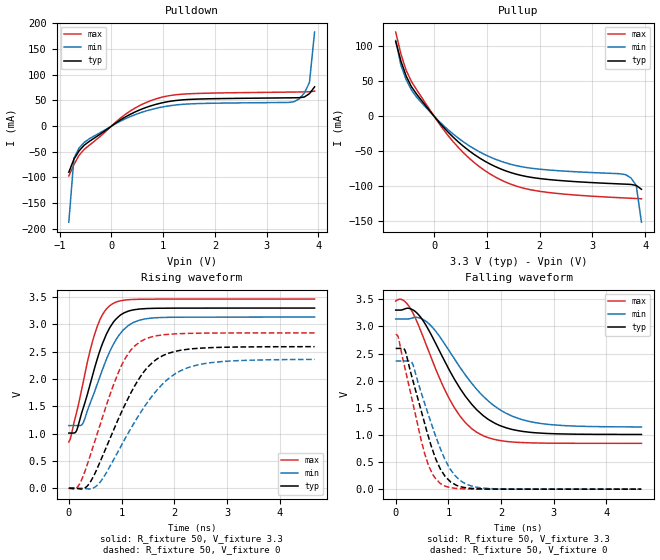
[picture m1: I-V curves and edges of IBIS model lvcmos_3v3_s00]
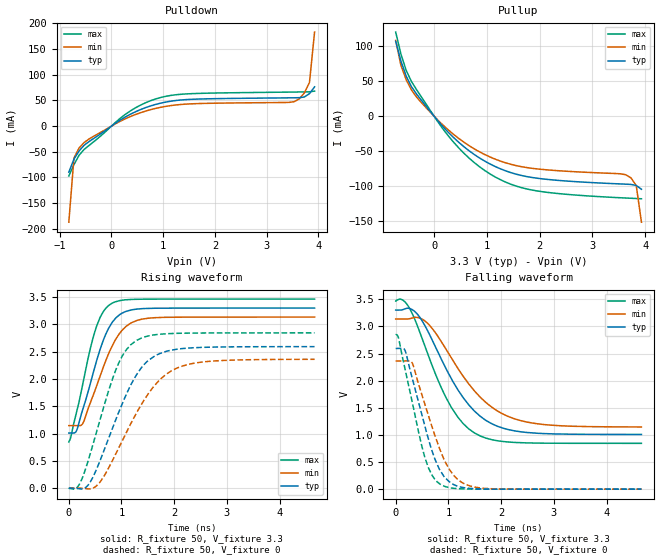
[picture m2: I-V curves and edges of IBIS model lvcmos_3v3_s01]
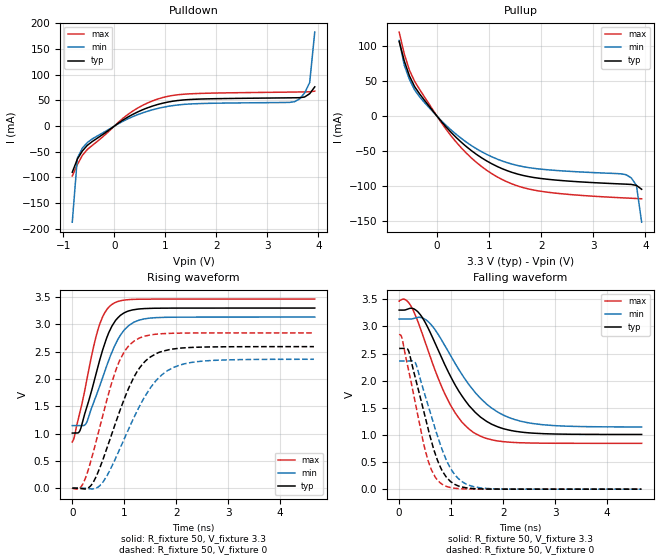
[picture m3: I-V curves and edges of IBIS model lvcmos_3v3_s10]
[IBIS ver]   4.1
[File name]   5p49v5907.ibs
[File Rev]   1.0
[Date]   May 27, 2015
[Source]   IDT
[Notes]   1. Temp typ=25C, min=85C, max=-40C
[Disclaimer]
READ THESE TERMS AND CONDITIONS CAREFULLY BEFORE USING THIS IBIS MODEL.  BY
USING THIS IBIS MODEL, YOU ARE ACCEPTING AND AGREEING TO THESE TERMS AND
CONDITIONS OF USE.
INTEGRATED DEVICE TECHNOLOGY, INC. ("IDT") HEREBY GRANTS THE USER OF THIS
IBIS MODEL ("USER") A NON-EXCLUSIVE, NONTRANSFERABLE LICENSE TO USE THIS
IBIS MODEL UNDER THE FOLLOWING TERMS: THE USER IS GRANTED THIS LICENSE ONLY
TO USE THE IBIS MODEL FOR DEMONSTRATION PURPOSES ONLY AND IS NOT GRANTED
RIGHTS TO SELL, COPY (EXCEPT AS NEEDED TO RUN THE IBIS MODEL), RENT, LEASE
OR SUB-LICENSE (EXCEPT FOR DEMONSTRATION) THE IBIS MODEL IN WHOLE OR IN
PART, OR IN MODIFIED FORM TO ANYONE. THE USER MAY MODIFY THE IBIS MODEL TO
SUIT ITS SPECIFIC APPLICATIONS, BUT  RIGHTS TO DERIVATIVE WORKS AND SUCH
MODIFICATIONS SHALL BELONG TO IDT.
THIS IBIS MODEL IS PROVIDED ON AN AS IS" BASIS AND IDT  MAKES ABSOLUTELY NO
WARRANTY WITH RESPECT TO THE INFORMATION CONTAINED HEREIN.  IDT DISCLAIMS
AND USER WAIVES ALL WARRANTIES, EXPRESS AND IMPLIED, INCLUDING WARRANTIES OF
MERCHANTABILITY AND FITNESS FOR A PARTICULAR PURPOSE.  THE ENTIRE RISK AS TO
QUALITY AND PERFORMANCE IS WITH THE USER  ACCORDINGLY, IN NO EVENT SHALL IDT
BE LIABLE FOR ANY DIRECT OR INDIRECT DAMAGES, WHETHER IN CONTRACT OR TORT,
INCLUDING ANY LOST PROFITS OR OTHER INCIDENTAL, CONSEQUENTIAL, EXEMPLARY, OR
PUNITIVE DAMAGES ARISING OUT OF THE USE OR APPLICATION OF THE  IBIS MODEL,
WHETHER OR NOT IDT HAD NOTICE OF SUCH DAMAGES.
IDT RESERVES THE RIGHT TO MAKE CHANGES WITHOUT NOTICE TO ANY PRODUCT HEREIN
TO IMPROVE RELIABILITY, FUNCTION, OR DESIGN. IDT DOES NOT CONVEY ANY LICENSE
UNDER PATENT RIGHTS OR ANY OTHER INTELLECTUAL PROPERTY RIGHTS, INCLUDING
THOSE OF THIRD PARTIES. IDT IS NOT OBLIGATED TO PROVIDE  MAINTENANCE OR
SUPPORT FOR THE LICENSED IBIS MODEL.
This model is for  vc5 IDT Programmable Clock
[Copyright]
Copyright 2002, Integrated Device Technology, Inc. All rights  reserved.
|History
|Rev 1.0 Created on May 27, 2015
|   Component IDT5p49v5907
[Component]   IDT5V49V5907
[Manufacturer]   Integrated Device Technology Inc.
[Package]
| Following package parameters are for the 24 pin QFN package
| variable   typ   min   max
R_pkg   72.4655m   58.886m   86.045m
L_pkg   1.47175nH   1.11650nH   1.77850nH
C_pkg   0.07747pF   0.07444pF   0.08050pF
[Pin]  signal_name   model_name
1   NC   NC
2   XOUT   NC
3   XIN/REF   input
4   VDDA   POWER
5   VDDO   POWER
6   OUT7   LP_HCSL
7   OUT7B   LP_HCSL
8   OUT6   LP_HCSL
9   OUT6B   LP_HCSL
10   SD/OE   input
11   SEL1/SDA   input
12   SEL0/SCL   input
13   VDD   POWER
14   VDDO   POWER
15   OUT5   LP_HCSL
16   OUT5B   LP_HCSL
17   OEB35   input
18   VDDO4   POWER
19   OUT4   UIO
20   OUT4B   UIO
21   NC   NC
22   NC   NC
23   OUT3B   LP_HCSL
24   OUT3   LP_HCSL
25   VDD_CORE   POWER
26   VDD   POWER
27   VDD   POWER
28   OUT2B   UIO
29   OUT2   UIO
30   VDDO2   POWER
31   OUT1B   UIO
32   OUT1   UIO
33   VDDO1   POWER
34   OEB67   input
35   NC   NC
36   VDDO   POWER
37   VDD   POWER
38   OEBUFFER   input
39   VDDO0   POWER
40   OUT0_SEL_I2C   UIOLVCMOS
[Diff Pin]  inv_pin  vdiff   tdelay_typ  tdelay_min  tdelay_max
|1   2   0.000V   0.000s   0.000s   0.000s
6   7   0.000V   0.000s   0.000s   0.000s
8   9   0.000V   0.000s   0.000s   0.000s
15   16   0.000V   0.000s   0.000s   0.000s
19   20   0.000V   0.000s   0.000s   0.000s
24   23   0.000V   0.000s   0.000s   0.000s
29   28   0.000V   0.000s   0.000s   0.000s
32   31   0.000V   0.000s   0.000s   0.000s
[Model Selector] UIO
lvcmos_3v3_s00 slew rate 00
lvcmos_3v3_s01 slew rate 01
lvcmos_3v3_s10 slew rate 10
lvcmos_3v3_s11 slew rate 11
lvcmos_2v5_s00 slew rate 00
lvcmos_2v5_s01 slew rate 01
lvcmos_2v5_s10 slew rate 10
lvcmos_2v5_s11 slew rate 11
lvcmos_1v8_s00 slew rate 00
lvcmos_1v8_s01 slew rate 01
lvcmos_1v8_s10 slew rate 10
lvcmos_1v8_s11 slew rate 11
hcsl_3v3 slew rate 11
hcsl_2v5 slew rate 11
lvds_3v3  slew rate 11
lvds_2v5  slew rate 11
lvpecl_3v3 slew rate 11
lvpecl_2v5 slew rate 11
[Model Selector] UIOLVCMOS
lvcmos_3v3_s00 slew rate 00
lvcmos_3v3_s01 slew rate 01
lvcmos_3v3_s10 slew rate 10
lvcmos_3v3_s11 slew rate 11
lvcmos_2v5_s00 slew rate 00
lvcmos_2v5_s01 slew rate 01
lvcmos_2v5_s10 slew rate 10
lvcmos_2v5_s11 slew rate 11
lvcmos_1v8_s00 slew rate 00
lvcmos_1v8_s01 slew rate 01
lvcmos_1v8_s10 slew rate 10
lvcmos_1v8_s11 slew rate 11
| Models and submodels in the file (20): lvcmos_3v3_s00 (Output), lvcmos_3v3_s01 (Output), lvcmos_3v3_s10 (Output), lvcmos_3v3_s11 (Output), lvcmos_2v5_s00 (Output), lvcmos_2v5_s01 (Output), lvcmos_2v5_s10 (Output), lvcmos_2v5_s11 (Output), lvcmos_1v8_s00 (Output), lvcmos_1v8_s01 (Output), lvcmos_1v8_s10 (Output), lvcmos_1v8_s11 (Output), hcsl_3v3 (Open_source), hcsl_2v5 (Open_source), lvds_3v3 (Output), lvds_2v5 (Output), lvpecl_3v3 (Output_ECL), lvpecl_2v5 (Output_ECL), LP_HCSL (Output), input (Input)
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|   Model LVCMOS_3V3
[Model]   lvcmos_3v3_s00
Model_type   Output
Polarity   Non-Inverting
|   typ   min   max
C_comp   2pF   1.5pF   2.5pF
Vmeas = 1.65V
Rref = 50
Cref = 0
Vref = 1.65V
|   typ   min   max
[Voltage range]   3.3V   3.135V   3.465V
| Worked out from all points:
|   slope of the pulldown table from 0 to 0.495 V, typ, clamps not added: 16.9 ohm
|   slope of the pullup table from 0 to 0.495 V, typ, clamps not added: 12.6 ohm
|   rising waveform, R_fixture 50, V_fixture 3.3: 20-80 % time 450ps typ, 507ps min, 388ps max; typ from 1.01 V to 3.3 V
|   falling waveform, R_fixture 50, V_fixture 3.3: 20-80 % time 857ps typ, 970ps min, 739ps max; typ from 3.3 V to 1.01 V
|   rising waveform, R_fixture 50, V_fixture 0: 20-80 % time 771ps typ, 936ps min, 618ps max; typ from 0 V to 2.59 V
|   falling waveform, R_fixture 50, V_fixture 0: 20-80 % time 472ps typ, 527ps min, 413ps max; typ from 2.59 V to 0 V
[Pulldown]
|Voltage   I (typ)   I (min)   I (max)
|Note, modeling breaks down at 250mA and above.  This is well beyond the functional   |
|operating range of the device.  Should this scenario occur, catastrophic failure and   |
|possible damage to the device and/or board is of higher concern than the I-V curve   |
|behavior.  The IBIS checker will flag currents in excess of 10A with warnings.  Lines   |
|with currents in excess of 0.35 A have been commented out.  The points still remain|
|available to the user if the user desires to use them.   |
|-3.30000e+00   -4.58626e+02   -3.98855e+02   -5.58913e+02
|-3.20100e+00   -4.38670e+02   -3.81813e+02   -5.34126e+02
|-3.10200e+00   -4.18718e+02   -3.64776e+02   -5.09343e+02
|-3.00300e+00   -3.98770e+02   -3.47745e+02   -4.84563e+02
|-2.90400e+00   -3.78827e+02   -3.30720e+02   -4.59787e+02
|-2.80500e+00   -3.58890e+02   -3.13701e+02   -4.35015e+02
|-2.70600e+00   -3.38959e+02   -2.96690e+02   -4.10248e+02
|-2.60700e+00   -3.19035e+02   -2.79688e+02   -3.85486e+02
|-2.50800e+00   -2.99119e+02   -2.62696e+02   -3.60731e+02
|-2.40900e+00   -2.79213e+02   -2.45715e+02   -3.35984e+02
|-2.31000e+00   -2.59319e+02   -2.28747e+02   -3.11245e+02
|-2.21100e+00   -2.39437e+02   -2.11796e+02   -2.86516e+02
|-2.11200e+00   -2.19572e+02   -1.94864e+02   -2.61800e+02
|-2.01300e+00   -1.99726e+02   -1.77955e+02   -2.37100e+02
|-1.91400e+00   -1.79905e+02   -1.61075e+02   -2.12419e+02
|-1.81500e+00   -1.60116e+02   -1.44233e+02   -1.87763e+02
|-1.71600e+00   -1.40369e+02   -1.27441e+02   -1.63140e+02
|-1.61700e+00   -1.20682e+02   -1.10717e+02   -1.38565e+02
|-1.51800e+00   -1.01080e+02   -9.40899e+01   -1.14061e+02
|-1.41900e+00   -8.16135e+01   -7.76121e+01   -8.96701e+01
|-1.32000e+00   -6.23864e+01   -6.13830e+01   -6.54941e+01
|-1.22100e+00   -4.36066e+01   -4.55730e+01   -4.17841e+01
|-1.12200e+00   -2.55446e+01   -3.03740e+01   -1.89497e+01
|-1.02300e+00   -8.13369e+00   -1.57511e+01   -1.01906e+00
|-9.24000e-01   -3.55892e-01   -2.38948e+00   -1.27879e-01
-825mV    -89.74mA   -186.9mA   -97.05mA
-726mV    -64.34mA   -62.46mA   -75.03mA
-627mV    -48.3mA    -42.65mA   -56.86mA
-528mV    -37.22mA   -31.89mA   -45.33mA
363mV     22.88mA    18.45mA    29.33mA
957mV     44.74mA    36.62mA    55.73mA
1.551V    52.05mA    43.3mA     63.04mA
3.531V    55.03mA    47.39mA    66.19mA
3.63V     55.21mA    52.95mA    66.32mA
3.729V    56.59mA    64.36mA    66.46mA
3.828V    63.02mA    84.81mA    66.64mA
3.927V    76.26mA    182.8mA    67.99mA
| 4.02600e+00   9.63336e-02   1.95544e+00   7.56685e-02
| 4.12500e+00   1.29319e-01   1.96109e+01   9.19025e-02
| 4.22400e+00   6.62462e-01   4.21550e+01   1.15435e-01
| 4.32300e+00   1.51637e+01   6.47670e+01   1.37492e-01
| 4.42200e+00   4.22442e+01   8.74545e+01   2.35006e-01
| 4.52100e+00   6.94172e+01   1.10195e+02   8.92943e+00
| 4.62000e+00   9.66780e+01   1.32968e+02   4.35589e+01
| 4.71900e+00   1.23991e+02   1.55761e+02   7.83218e+01
| 4.81800e+00   1.51333e+02   1.78569e+02   1.13180e+02
| 4.91700e+00   1.78693e+02   2.01386e+02   1.48085e+02
| 5.01600e+00   2.06065e+02   2.24210e+02   1.83014e+02
| 5.11500e+00   2.33446e+02   2.47041e+02   2.17958e+02
| 5.21400e+00   2.60834e+02   2.69877e+02   2.52912e+02
| 5.31300e+00   2.88228e+02   2.92717e+02   2.87874e+02
| 5.41200e+00   3.15625e+02   3.15560e+02   3.22841e+02
| 5.51100e+00   3.43027e+02   3.38407e+02   3.57813e+02
| 5.61000e+00   3.70432e+02   3.61256e+02   3.92789e+02
| 5.70900e+00   3.97841e+02   3.84108e+02   4.27769e+02
| 5.80800e+00   4.25252e+02   4.06963e+02   4.62752e+02
| 5.90700e+00   4.52666e+02   4.29821e+02   4.97738e+02
| 6.00600e+00   4.80082e+02   4.52680e+02   5.32727e+02
| 6.10500e+00   5.07501e+02   4.75543e+02   5.67718e+02
| 6.20400e+00   5.34922e+02   4.98407e+02   6.02711e+02
| 6.30300e+00   5.62345e+02   5.21273e+02   6.37705e+02
| 6.40200e+00   5.89770e+02   5.44142e+02   6.72701e+02
| 6.50100e+00   6.17197e+02   5.67013e+02   7.07699e+02
| 6.60000e+00   6.44626e+02   5.89886e+02   7.42698e+02
[Pullup]
|Voltage   I (typ)   I (min)   I (max)
|Note, modeling breaks down at 250mA and above.  This is well beyond the functional   |
|operating range of the device.  Should this scenario occur, catastrophic failure and   |
|possible damage to the device and/or board is of higher concern than the I-V curve   |
|behavior.  The IBIS checker will flag currents in excess of 10A with warnings.  Lines   |
|with currents in excess of 0.35 A have been commented out.  The points still remain|
|available to the user if the user desires to use them.   |
|-3.30000e+00   6.44680e+02   5.51825e+02   8.01095e+02
|-3.20100e+00   6.17254e+02   5.28958e+02   7.66095e+02
|-3.10200e+00   5.89830e+02   5.06093e+02   7.31096e+02
|-3.00300e+00   5.62407e+02   4.83230e+02   6.96098e+02
|-2.90400e+00   5.34987e+02   4.60368e+02   6.61102e+02
|-2.80500e+00   5.07568e+02   4.37509e+02   6.26108e+02
|-2.70600e+00   4.80150e+02   4.14651e+02   5.91115e+02
|-2.60700e+00   4.52735e+02   3.91796e+02   5.56124e+02
|-2.50800e+00   4.25322e+02   3.68942e+02   5.21136e+02
|-2.40900e+00   3.97911e+02   3.46091e+02   4.86149e+02
|-2.31000e+00   3.70503e+02   3.23243e+02   4.51165e+02
|-2.21100e+00   3.43097e+02   3.00397e+02   4.16183e+02
|-2.11200e+00   3.15694e+02   2.77554e+02   3.81204e+02
|-2.01300e+00   2.88295e+02   2.54715e+02   3.46229e+02
|-1.91400e+00   2.60900e+02   2.31881e+02   3.11257e+02
|-1.81500e+00   2.33510e+02   2.09052e+02   2.76290e+02
|-1.71600e+00   2.06127e+02   1.86229e+02   2.41329e+02
|-1.61700e+00   1.78751e+02   1.63415e+02   2.06375e+02
|-1.51800e+00   1.51388e+02   1.40613e+02   1.71432e+02
|-1.41900e+00   1.24042e+02   1.17829e+02   1.36506e+02
|-1.32000e+00   9.67252e+01   9.50724e+01   1.01609e+02
|-1.22100e+00   6.94599e+01   7.23604e+01   6.67700e+01
|-1.12200e+00   4.22820e+01   4.97173e+01   3.20469e+01
|-1.02300e+00   1.51962e+01   2.71494e+01   2.11287e+00
|-9.24000e-01   6.89030e-01   5.34223e+00   1.97623e-01
|-8.25000e-01   1.48916e-01   3.54714e-01   1.54087e-01
-726mV    106.9mA    108.2mA    120.1mA
-627mV    78.63mA    72.64mA    88.74mA
-528mV    57.36mA    52.3mA     65.5mA
-330mV    31.45mA    27.24mA    37.82mA
363mV     -30.02mA   -25.58mA   -36.52mA
957mV     -64.05mA   -54.65mA   -77.43mA
1.353V    -77.99mA   -66.51mA   -94.06mA
1.848V    -87.45mA   -74.38mA   -105.4mA
3.63V     -97.08mA   -83.63mA   -116.9mA
3.729V    -97.47mA   -88.18mA   -117.2mA
3.828V    -98.9mA    -99mA      -117.5mA
3.927V    -104.4mA   -151.4mA   -117.9mA
| 4.02600e+00   -1.15410e-01   -9.65481e-01   -1.19366e-01
| 4.12500e+00   -1.36603e-01   -1.09884e+01   -1.26324e-01
| 4.22400e+00   -3.99361e-01   -2.54841e+01   -1.40663e-01
| 4.32300e+00   -8.17474e+00   -4.04654e+01   -1.58277e-01
| 4.42200e+00   -2.55843e+01   -5.60873e+01   -2.17491e-01
| 4.52100e+00   -4.36450e+01   -7.21990e+01   -4.28595e+00
| 4.62000e+00   -6.24226e+01   -8.86071e+01   -2.64922e+01
| 4.71900e+00   -8.16508e+01   -1.05189e+02   -4.96573e+01
| 4.81800e+00   -1.01115e+02   -1.21884e+02   -7.35635e+01
| 4.91700e+00   -1.20715e+02   -1.38656e+02   -9.78285e+01
| 5.01600e+00   -1.40403e+02   -1.55482e+02   -1.22263e+02
| 5.11500e+00   -1.60149e+02   -1.72350e+02   -1.46794e+02
| 5.21400e+00   -1.79938e+02   -1.89250e+02   -1.71387e+02
| 5.31300e+00   -1.99760e+02   -2.06175e+02   -1.96022e+02
| 5.41200e+00   -2.19606e+02   -2.23121e+02   -2.20688e+02
| 5.51100e+00   -2.39472e+02   -2.40084e+02   -2.45378e+02
| 5.61000e+00   -2.59355e+02   -2.57061e+02   -2.70086e+02
| 5.70900e+00   -2.79251e+02   -2.74051e+02   -2.94808e+02
| 5.80800e+00   -2.99159e+02   -2.91052e+02   -3.19543e+02
| 5.90700e+00   -3.19077e+02   -3.08062e+02   -3.44288e+02
| 6.00600e+00   -3.39003e+02   -3.25080e+02   -3.69042e+02
| 6.10500e+00   -3.58937e+02   -3.42106e+02   -3.93803e+02
| 6.20400e+00   -3.78878e+02   -3.59138e+02   -4.18571e+02
| 6.30300e+00   -3.98826e+02   -3.76177e+02   -4.43346e+02
| 6.40200e+00   -4.18779e+02   -3.93221e+02   -4.68125e+02
| 6.50100e+00   -4.38737e+02   -4.10271e+02   -4.92910e+02
| 6.60000e+00   -4.58699e+02   -4.27325e+02   -5.17700e+02
[Ramp]
|   typ   min   max
dV/dt_r   1.566/0.774n   1.425/0.94n   1.718/0.621n
dV/dt_f   1.396/0.866n   1.212/0.979n   1.595/0.746n
R_load =   50
[Rising Waveform]
R_fixture = 50
V_fixture = 3.3   |Vcc_typ
V_fixture_min = 3.135 |Vcc_min
V_fixture_max = 3.465 |Vcc_max
C_fixture = 0.0p
| Time   typ   min   max
| 0.00000e+00   1.00813e+00   1.14515e+00   8.44568e-01
| 2.69541e-12   1.00813e+00   1.14515e+00   8.44568e-01
| 4.88539e-12   1.00813e+00   1.14515e+00   8.44568e-01
| 5.15560e-12   1.00813e+00   1.14515e+00   8.44568e-01
| 8.43814e-12   1.00813e+00   1.14515e+00   8.44568e-01
| 1.48885e-11   1.00813e+00   1.14515e+00   8.44568e-01
| 1.56443e-11   1.00813e+00   1.14515e+00   8.44568e-01
| 2.89352e-11   1.00813e+00   1.14515e+00   8.44568e-01
| 4.35521e-11   1.00813e+00   1.14515e+00   8.44568e-01
| 4.98146e-11   1.00813e+00   1.14515e+00   8.44568e-01
| 5.87208e-11   1.00813e+00   1.14515e+00   8.44568e-01
| 7.00000e-11   1.00813e+00   1.14515e+00   8.44568e-01
| 7.43355e-11   1.00813e+00   1.14515e+00   8.44568e-01
| 7.98941e-11   1.00813e+00   1.14515e+00   8.44568e-01
| 8.04812e-11   1.00813e+00   1.14515e+00   8.44568e-01
| 8.54765e-11   1.00813e+00   1.14515e+00   8.44568e-01
| 9.54712e-11   1.00813e+00   1.14515e+00   8.44568e-01
| 9.66941e-11   1.00813e+00   1.14515e+00   8.44568e-01
| 1.09694e-10   1.00813e+00   1.14515e+00   8.44568e-01
| 1.16904e-10   1.00813e+00   1.14515e+00   8.44568e-01
| 1.22050e-10   1.00813e+00   1.14515e+00   8.44568e-01
| 1.33756e-10   1.00813e+00   1.14515e+00   8.44568e-01
| 1.42319e-10   1.00813e+00   1.14515e+00   8.44568e-01
| 1.49876e-10   1.00813e+00   1.14515e+00   8.44568e-01
| 1.59675e-10   1.00813e+00   1.14515e+00   8.44568e-01
| 1.71924e-10   1.00813e+00   1.14515e+00   8.44568e-01
| 1.80502e-10   1.00813e+00   1.14515e+00   8.44568e-01
| 1.93342e-10   1.00813e+00   1.14515e+00   8.44568e-01
| 2.03187e-10   1.00813e+00   1.14515e+00   8.44568e-01
| 2.12788e-10   1.00813e+00   1.14515e+00   8.44568e-01
| 2.20117e-10   1.00813e+00   1.14515e+00   8.44568e-01
| 2.25959e-10   1.00813e+00   1.14515e+00   8.44568e-01
| 2.28188e-10   1.00813e+00   1.14515e+00   8.44568e-01
| 2.36412e-10   1.00813e+00   1.14515e+00   8.44568e-01
| 2.43714e-10   1.00813e+00   1.14515e+00   8.44568e-01
| 2.46567e-10   1.00813e+00   1.14515e+00   8.44568e-01
| 2.54564e-10   1.00813e+00   1.14515e+00   8.44568e-01
| 2.64894e-10   1.00813e+00   1.14515e+00   8.44568e-01
| 2.65919e-10   1.00813e+00   1.14515e+00   8.44568e-01
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0s        1.008V     1.145V     844.6mV
34.71ps   1.008V     1.145V     923.1mV
154.3ps   1.071V     1.145V     1.413V
275.2ps   1.472V     1.202V     1.956V
479.5ps   2.168V     1.745V     2.789V
635.5ps   2.641V     2.166V     3.174V
823.7ps   3.01V      2.596V     3.375V
1.129ns   3.244V     2.981V     3.453V
1.433ns   3.289V     3.099V     3.463V
4.662ns   3.3V       3.135V     3.465V
[Falling Waveform]
R_fixture = 50
V_fixture = 3.3   |Vcc_typ
V_fixture_min = 3.135 |Vcc_min
V_fixture_max = 3.465 |Vcc_max
C_fixture = 0.0p
| Time   typ   min   max
| 0.00000e+00   3.30000e+00   3.13500e+00   3.46500e+00
| 2.69541e-12   3.30000e+00   3.13500e+00   3.46500e+00
| 4.88539e-12   3.30000e+00   3.13500e+00   3.46500e+00
| 5.15560e-12   3.30000e+00   3.13500e+00   3.46500e+00
| 8.43814e-12   3.30000e+00   3.13500e+00   3.46500e+00
| 1.48885e-11   3.30000e+00   3.13500e+00   3.46500e+00
| 1.56443e-11   3.30000e+00   3.13500e+00   3.46500e+00
| 2.89352e-11   3.30000e+00   3.13500e+00   3.46500e+00
| 4.35521e-11   3.30000e+00   3.13500e+00   3.46500e+00
| 4.98146e-11   3.30000e+00   3.13500e+00   3.46500e+00
| 5.87207e-11   3.30000e+00   3.13500e+00   3.46500e+00
| 7.00000e-11   3.30000e+00   3.13500e+00   3.46500e+00
| 7.43355e-11   3.30000e+00   3.13500e+00   3.46500e+00
| 7.98941e-11   3.30000e+00   3.13500e+00   3.46500e+00
| 8.04812e-11   3.30000e+00   3.13500e+00   3.46500e+00
| 8.54765e-11   3.30000e+00   3.13500e+00   3.46500e+00
| 9.54712e-11   3.30000e+00   3.13500e+00   3.46500e+00
| 9.66941e-11   3.30000e+00   3.13500e+00   3.46500e+00
| 1.09694e-10   3.30000e+00   3.13500e+00   3.46500e+00
| 1.16904e-10   3.30000e+00   3.13500e+00   3.46500e+00
| 1.22050e-10   3.30000e+00   3.13500e+00   3.46500e+00
| 1.33756e-10   3.30000e+00   3.13500e+00   3.46500e+00
| 1.42318e-10   3.30000e+00   3.13500e+00   3.46500e+00
| 1.49875e-10   3.30000e+00   3.13500e+00   3.46500e+00
| 1.59673e-10   3.30000e+00   3.13500e+00   3.46500e+00
| 1.72937e-10   3.30000e+00   3.13500e+00   3.46500e+00
| 1.80499e-10   3.30000e+00   3.13500e+00   3.46500e+00
| 1.94084e-10   3.30000e+00   3.13500e+00   3.46500e+00
| 2.03953e-10   3.30000e+00   3.13500e+00   3.46500e+00
| 2.17182e-10   3.30000e+00   3.13500e+00   3.46500e+00
| 2.22997e-10   3.30000e+00   3.13500e+00   3.46500e+00
| 2.32435e-10   3.30000e+00   3.13500e+00   3.46500e+00
| 2.41161e-10   3.30000e+00   3.13500e+00   3.46500e+00
| 2.46386e-10   3.30000e+00   3.13500e+00   3.46500e+00
| 2.56120e-10   3.30000e+00   3.13500e+00   3.46500e+00
| 2.57140e-10   3.30000e+00   3.13500e+00   3.46500e+00
| 2.66989e-10   3.30000e+00   3.13500e+00   3.46500e+00
| 2.77410e-10   3.30000e+00   3.13500e+00   3.46500e+00
| 2.83433e-10   3.30000e+00   3.13500e+00   3.46500e+00
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0s        3.3V       3.135V     3.465V
120.3ps   3.304V     3.135V     3.493V
247.8ps   3.333V     3.138V     3.377V
425ps     3.225V     3.162V     3.038V
624.4ps   2.937V     3.054V     2.545V
1.111ns   2.034V     2.407V     1.506V
1.539ns   1.462V     1.838V     1.048V
1.979ns   1.171V     1.463V     896.3mV
2.515ns   1.052V     1.252V     854.4mV
4.666ns   1.008V     1.146V     844.6mV
[Rising Waveform]
R_fixture = 50
V_fixture = 0
C_fixture = 0.0p
| Time   typ   min   max
| 0.00000e+00   2.38922e-08   6.04307e-08   3.04013e-08
| 2.76195e-12   2.38928e-08   6.04313e-08   3.04019e-08
| 5.02196e-12   2.38933e-08   6.04317e-08   3.04024e-08
| 8.43814e-12   2.38939e-08   6.04323e-08   3.04029e-08
| 1.48885e-11   2.38940e-08   6.04329e-08   3.04024e-08
| 2.82261e-11   2.38916e-08   6.04313e-08   3.03997e-08
| 2.96292e-11   2.38914e-08   6.04311e-08   3.03993e-08
| 4.65264e-11   2.38885e-08   6.04278e-08   3.03985e-08
| 5.82632e-11   2.38858e-08   6.04236e-08   3.03966e-08
| 5.99073e-11   2.38849e-08   6.04221e-08   3.03962e-08
| 7.43093e-11   2.38731e-08   6.04054e-08   3.03887e-08
| 7.44096e-11   2.38730e-08   6.04053e-08   3.03887e-08
| 8.01162e-11   2.38724e-08   6.03982e-08   3.03965e-08
| 8.50865e-11   2.38893e-08   6.04041e-08   3.04290e-08
| 8.58855e-11   2.38922e-08   6.04086e-08   3.04412e-08
| 9.61972e-11   2.40299e-08   6.05121e-08   3.05978e-08
| 1.07592e-10   2.42393e-08   6.07310e-08   3.07509e-08
| 1.10532e-10   2.42814e-08   6.07875e-08   3.07287e-08
| 1.20263e-10   2.43168e-08   6.09006e-08   3.05636e-08
| 1.31586e-10   2.39714e-08   6.07198e-08   3.01694e-08
| 1.35499e-10   2.37749e-08   6.06371e-08   2.99415e-08
| 1.46539e-10   2.29494e-08   5.97382e-08   2.91160e-08
| 1.55369e-10   2.17459e-08   5.85776e-08   2.82197e-08
| 1.63542e-10   2.08213e-08   5.72547e-08   2.77163e-08
| 1.77096e-10   1.96380e-08   5.55739e-08   2.77900e-08
| 1.86474e-10   2.06626e-08   5.56638e-08   2.88594e-08
| 1.98457e-10   2.24638e-08   5.66917e-08   3.14335e-08
| 2.09942e-10   2.48230e-08   5.90292e-08   3.38303e-08
| 2.15324e-10   2.58385e-08   6.01248e-08   3.48209e-08
| 2.20167e-10   2.67523e-08   6.09774e-08   3.56015e-08
| 2.27556e-10   2.81666e-08   6.22968e-08   3.65293e-08
| 2.34644e-10   2.94091e-08   6.36265e-08   3.66031e-08
| 2.36605e-10   2.97316e-08   6.40403e-08   3.66235e-08
| 2.44185e-10   3.03330e-08   6.55688e-08   3.54311e-08
| 2.54086e-10   3.02460e-08   6.61635e-08   3.24030e-08
| 2.55652e-10   3.01885e-08   6.60924e-08   3.18824e-08
| 2.65464e-10   2.87011e-08   6.51928e-08   2.86958e-08
| 2.76364e-10   2.59383e-08   6.40745e-08   2.65085e-08
| 2.78193e-10   2.54665e-08   6.38562e-08   2.63589e-08
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0s        23.89nV    60.43nV    30.4nV
191.1ps   -13.44mV   129.7uV    54.48mV
415.8ps   124mV      -13.01mV   625.4mV
623.1ps   548.9mV    147.1mV    1.254V
939.4ps   1.267V     680mV      2.117V
1.156ns   1.708V     1.059V     2.505V
1.348ns   2.027V     1.367V     2.681V
1.787ns   2.43V      1.916V     2.809V
2.339ns   2.554V     2.232V     2.838V
4.662ns   2.593V     2.359V     2.845V
[Falling Waveform]
R_fixture = 50
V_fixture = 0
C_fixture = 0.0p
| Time   typ   min   max
| 0.00000e+00   2.59298e+00   2.36182e+00   2.84510e+00
| 7.32301e-10   2.59297e+00   2.36182e+00   2.84511e+00
| 7.45695e-10   2.59297e+00   2.36182e+00   2.84508e+00
| 7.56189e-10   2.59297e+00   2.36182e+00   2.84504e+00
| 7.64187e-10   2.59297e+00   2.36182e+00   2.84501e+00
| 7.77879e-10   2.59298e+00   2.36182e+00   2.84495e+00
| 7.83323e-10   2.59298e+00   2.36182e+00   2.84491e+00
| 7.94399e-10   2.59298e+00   2.36182e+00   2.84472e+00
| 7.99287e-10   2.59298e+00   2.36182e+00   2.84484e+00
| 8.04717e-10   2.59298e+00   2.36182e+00   2.84527e+00
| 8.14850e-10   2.59298e+00   2.36182e+00   2.84673e+00
| 8.19261e-10   2.59298e+00   2.36182e+00   2.84748e+00
| 8.29192e-10   2.59298e+00   2.36182e+00   2.84897e+00
| 8.30495e-10   2.59298e+00   2.36182e+00   2.84912e+00
| 8.41433e-10   2.59297e+00   2.36182e+00   2.84930e+00
| 8.47210e-10   2.59297e+00   2.36182e+00   2.84828e+00
| 8.58618e-10   2.59294e+00   2.36182e+00   2.84222e+00
| 8.63453e-10   2.59293e+00   2.36182e+00   2.83856e+00
| 8.70885e-10   2.59291e+00   2.36182e+00   2.82897e+00
| 8.82012e-10   2.59289e+00   2.36182e+00   2.80438e+00
| 8.91483e-10   2.59287e+00   2.36182e+00   2.77076e+00
| 8.98876e-10   2.59284e+00   2.36182e+00   2.73808e+00
| 9.04944e-10   2.59279e+00   2.36182e+00   2.71030e+00
| 9.12619e-10   2.59275e+00   2.36182e+00   2.67316e+00
| 9.19838e-10   2.59289e+00   2.36182e+00   2.63632e+00
| 9.26265e-10   2.59328e+00   2.36182e+00   2.60345e+00
| 9.32501e-10   2.59385e+00   2.36182e+00   2.57143e+00
| 9.39357e-10   2.59458e+00   2.36181e+00   2.53748e+00
| 9.43037e-10   2.59498e+00   2.36181e+00   2.51926e+00
| 9.52526e-10   2.59582e+00   2.36181e+00   2.47546e+00
| 9.56341e-10   2.59595e+00   2.36181e+00   2.45847e+00
| 9.64823e-10   2.59585e+00   2.36179e+00   2.42128e+00
| 9.70148e-10   2.59508e+00   2.36178e+00   2.39878e+00
| 9.77630e-10   2.59321e+00   2.36177e+00   2.36729e+00
| 9.82631e-10   2.59094e+00   2.36176e+00   2.34653e+00
| 9.89329e-10   2.58680e+00   2.36175e+00   2.31872e+00
| 9.97524e-10   2.57966e+00   2.36174e+00   2.28462e+00
| 1.00394e-09   2.57078e+00   2.36173e+00   2.25795e+00
| 1.01210e-09   2.55458e+00   2.36172e+00   2.22378e+00
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0s        2.593V     2.362V     2.845V
47.92ps   2.593V     2.362V     2.804V
169.8ps   2.571V     2.362V     2.258V
309ps     2.063V     2.332V     1.656V
482.9ps   1.445V     1.783V     905.2mV
624.2ps   958.6mV    1.36V      434.3mV
847.8ps   371.4mV    743.3mV    103.8mV
1.113ns   93.12mV    264.4mV    16.96mV
1.53ns    8.102mV    37.41mV    1.012mV
4.662ns   -1.039uV   -794nV     -867.7nV
[Model]   lvcmos_3v3_s01
Model_type   Output
Polarity   Non-Inverting
|   typ   min   max
C_comp   2pF   1.5pF   2.5pF
Vmeas = 1.65V
Rref = 50
Cref = 0
Vref = 1.65V
|   typ   min   max
[Voltage range]   3.3V   3.135V   3.465V
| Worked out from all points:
|   slope of the pulldown table from 0 to 0.495 V, typ, clamps not added: 16.9 ohm
|   slope of the pullup table from 0 to 0.495 V, typ, clamps not added: 12.6 ohm
|   rising waveform, R_fixture 50, V_fixture 3.3: 20-80 % time 438ps typ, 496ps min, 375ps max; typ from 1.01 V to 3.3 V
|   falling waveform, R_fixture 50, V_fixture 3.3: 20-80 % time 821ps typ, 925ps min, 710ps max; typ from 3.3 V to 1.01 V
|   rising waveform, R_fixture 50, V_fixture 0: 20-80 % time 684ps typ, 824ps min, 552ps max; typ from 0 V to 2.59 V
|   falling waveform, R_fixture 50, V_fixture 0: 20-80 % time 454ps typ, 508ps min, 394ps max; typ from 2.59 V to 0 V
[Pulldown]
|Voltage   I (typ)   I (min)   I (max)
|Note, modeling breaks down at 250mA and above.  This is well beyond the functional   |
|operating range of the device.  Should this scenario occur, catastrophic failure and   |
|possible damage to the device and/or board is of higher concern than the I-V curve   |
|behavior.  The IBIS checker will flag currents in excess of 10A with warnings.  Lines   |
|with currents in excess of 0.35 A have been commented out.  The points still remain|
|available to the user if the user desires to use them.   |
|-3.30000e+00   -4.58626e+02   -3.98855e+02   -5.58913e+02
|-3.20100e+00   -4.38670e+02   -3.81813e+02   -5.34126e+02
|-3.10200e+00   -4.18718e+02   -3.64776e+02   -5.09343e+02
|-3.00300e+00   -3.98770e+02   -3.47745e+02   -4.84563e+02
|-2.90400e+00   -3.78827e+02   -3.30720e+02   -4.59787e+02
|-2.80500e+00   -3.58890e+02   -3.13701e+02   -4.35015e+02
|-2.70600e+00   -3.38959e+02   -2.96690e+02   -4.10248e+02
|-2.60700e+00   -3.19035e+02   -2.79688e+02   -3.85486e+02
|-2.50800e+00   -2.99119e+02   -2.62696e+02   -3.60731e+02
|-2.40900e+00   -2.79213e+02   -2.45715e+02   -3.35984e+02
|-2.31000e+00   -2.59319e+02   -2.28747e+02   -3.11245e+02
|-2.21100e+00   -2.39437e+02   -2.11796e+02   -2.86516e+02
|-2.11200e+00   -2.19572e+02   -1.94864e+02   -2.61800e+02
|-2.01300e+00   -1.99726e+02   -1.77955e+02   -2.37100e+02
|-1.91400e+00   -1.79905e+02   -1.61075e+02   -2.12419e+02
|-1.81500e+00   -1.60116e+02   -1.44233e+02   -1.87763e+02
|-1.71600e+00   -1.40369e+02   -1.27441e+02   -1.63140e+02
|-1.61700e+00   -1.20682e+02   -1.10717e+02   -1.38565e+02
|-1.51800e+00   -1.01080e+02   -9.40899e+01   -1.14061e+02
|-1.41900e+00   -8.16135e+01   -7.76121e+01   -8.96701e+01
|-1.32000e+00   -6.23864e+01   -6.13830e+01   -6.54941e+01
|-1.22100e+00   -4.36066e+01   -4.55730e+01   -4.17841e+01
|-1.12200e+00   -2.55446e+01   -3.03740e+01   -1.89497e+01
|-1.02300e+00   -8.13369e+00   -1.57511e+01   -1.01906e+00
|-9.24000e-01   -3.55892e-01   -2.38948e+00   -1.27879e-01
-825mV    -89.74mA   -186.9mA   -97.05mA
-726mV    -64.34mA   -62.46mA   -75.03mA
-627mV    -48.3mA    -42.65mA   -56.86mA
-528mV    -37.22mA   -31.89mA   -45.33mA
363mV     22.88mA    18.45mA    29.33mA
957mV     44.74mA    36.62mA    55.73mA
1.551V    52.05mA    43.3mA     63.04mA
3.531V    55.03mA    47.39mA    66.19mA
3.63V     55.21mA    52.95mA    66.32mA
3.729V    56.59mA    64.36mA    66.46mA
3.828V    63.02mA    84.81mA    66.64mA
3.927V    76.26mA    182.8mA    67.99mA
| 4.02600e+00   9.63336e-02   1.95544e+00   7.56685e-02
| 4.12500e+00   1.29319e-01   1.96109e+01   9.19025e-02
| 4.22400e+00   6.62462e-01   4.21550e+01   1.15435e-01
| 4.32300e+00   1.51637e+01   6.47670e+01   1.37492e-01
| 4.42200e+00   4.22442e+01   8.74545e+01   2.35006e-01
| 4.52100e+00   6.94172e+01   1.10195e+02   8.92943e+00
| 4.62000e+00   9.66780e+01   1.32968e+02   4.35589e+01
| 4.71900e+00   1.23991e+02   1.55761e+02   7.83218e+01
| 4.81800e+00   1.51333e+02   1.78569e+02   1.13180e+02
| 4.91700e+00   1.78693e+02   2.01386e+02   1.48085e+02
| 5.01600e+00   2.06065e+02   2.24210e+02   1.83014e+02
| 5.11500e+00   2.33446e+02   2.47041e+02   2.17958e+02
| 5.21400e+00   2.60834e+02   2.69877e+02   2.52912e+02
| 5.31300e+00   2.88228e+02   2.92717e+02   2.87874e+02
| 5.41200e+00   3.15625e+02   3.15560e+02   3.22841e+02
| 5.51100e+00   3.43027e+02   3.38407e+02   3.57813e+02
| 5.61000e+00   3.70432e+02   3.61256e+02   3.92789e+02
| 5.70900e+00   3.97841e+02   3.84108e+02   4.27769e+02
| 5.80800e+00   4.25252e+02   4.06963e+02   4.62752e+02
| 5.90700e+00   4.52666e+02   4.29821e+02   4.97738e+02
| 6.00600e+00   4.80082e+02   4.52680e+02   5.32727e+02
| 6.10500e+00   5.07501e+02   4.75543e+02   5.67718e+02
| 6.20400e+00   5.34922e+02   4.98407e+02   6.02711e+02
| 6.30300e+00   5.62345e+02   5.21273e+02   6.37705e+02
| 6.40200e+00   5.89770e+02   5.44142e+02   6.72701e+02
| 6.50100e+00   6.17197e+02   5.67013e+02   7.07699e+02
| 6.60000e+00   6.44626e+02   5.89886e+02   7.42698e+02
[Pullup]
|Voltage   I (typ)   I (min)   I (max)
|Note, modeling breaks down at 250mA and above.  This is well beyond the functional   |
|operating range of the device.  Should this scenario occur, catastrophic failure and   |
|possible damage to the device and/or board is of higher concern than the I-V curve   |
|behavior.  The IBIS checker will flag currents in excess of 10A with warnings.  Lines   |
|with currents in excess of 0.35 A have been commented out.  The points still remain|
|available to the user if the user desires to use them.   |
|-3.30000e+00   6.44680e+02   5.51825e+02   8.01095e+02
|-3.20100e+00   6.17254e+02   5.28958e+02   7.66095e+02
|-3.10200e+00   5.89830e+02   5.06093e+02   7.31096e+02
|-3.00300e+00   5.62407e+02   4.83230e+02   6.96098e+02
|-2.90400e+00   5.34987e+02   4.60368e+02   6.61102e+02
|-2.80500e+00   5.07568e+02   4.37509e+02   6.26108e+02
|-2.70600e+00   4.80150e+02   4.14651e+02   5.91115e+02
|-2.60700e+00   4.52735e+02   3.91796e+02   5.56124e+02
|-2.50800e+00   4.25322e+02   3.68942e+02   5.21136e+02
|-2.40900e+00   3.97911e+02   3.46091e+02   4.86149e+02
|-2.31000e+00   3.70503e+02   3.23243e+02   4.51165e+02
|-2.21100e+00   3.43097e+02   3.00397e+02   4.16183e+02
|-2.11200e+00   3.15694e+02   2.77554e+02   3.81204e+02
|-2.01300e+00   2.88295e+02   2.54715e+02   3.46229e+02
|-1.91400e+00   2.60900e+02   2.31881e+02   3.11257e+02
|-1.81500e+00   2.33510e+02   2.09052e+02   2.76290e+02
|-1.71600e+00   2.06127e+02   1.86229e+02   2.41329e+02
|-1.61700e+00   1.78751e+02   1.63415e+02   2.06375e+02
|-1.51800e+00   1.51388e+02   1.40613e+02   1.71432e+02
|-1.41900e+00   1.24042e+02   1.17829e+02   1.36506e+02
|-1.32000e+00   9.67252e+01   9.50724e+01   1.01609e+02
|-1.22100e+00   6.94599e+01   7.23604e+01   6.67700e+01
|-1.12200e+00   4.22820e+01   4.97173e+01   3.20469e+01
|-1.02300e+00   1.51962e+01   2.71494e+01   2.11287e+00
|-9.24000e-01   6.89030e-01   5.34223e+00   1.97623e-01
|-8.25000e-01   1.48916e-01   3.54714e-01   1.54087e-01
-726mV    106.9mA    108.2mA    120.1mA
-627mV    78.63mA    72.64mA    88.74mA
-528mV    57.36mA    52.3mA     65.5mA
-330mV    31.45mA    27.24mA    37.82mA
363mV     -30.02mA   -25.58mA   -36.52mA
957mV     -64.05mA   -54.65mA   -77.43mA
1.353V    -77.99mA   -66.51mA   -94.06mA
1.848V    -87.45mA   -74.38mA   -105.4mA
3.63V     -97.08mA   -83.63mA   -116.9mA
3.729V    -97.47mA   -88.18mA   -117.2mA
3.828V    -98.9mA    -99mA      -117.5mA
3.927V    -104.4mA   -151.4mA   -117.9mA
| 4.02600e+00   -1.15410e-01   -9.65481e-01   -1.19366e-01
| 4.12500e+00   -1.36603e-01   -1.09884e+01   -1.26324e-01
| 4.22400e+00   -3.99361e-01   -2.54841e+01   -1.40663e-01
| 4.32300e+00   -8.17474e+00   -4.04654e+01   -1.58277e-01
| 4.42200e+00   -2.55843e+01   -5.60873e+01   -2.17491e-01
| 4.52100e+00   -4.36450e+01   -7.21990e+01   -4.28595e+00
| 4.62000e+00   -6.24226e+01   -8.86071e+01   -2.64922e+01
| 4.71900e+00   -8.16508e+01   -1.05189e+02   -4.96573e+01
| 4.81800e+00   -1.01115e+02   -1.21884e+02   -7.35635e+01
| 4.91700e+00   -1.20715e+02   -1.38656e+02   -9.78285e+01
| 5.01600e+00   -1.40403e+02   -1.55482e+02   -1.22263e+02
| 5.11500e+00   -1.60149e+02   -1.72350e+02   -1.46794e+02
| 5.21400e+00   -1.79938e+02   -1.89250e+02   -1.71387e+02
| 5.31300e+00   -1.99760e+02   -2.06175e+02   -1.96022e+02
| 5.41200e+00   -2.19606e+02   -2.23121e+02   -2.20688e+02
| 5.51100e+00   -2.39472e+02   -2.40084e+02   -2.45378e+02
| 5.61000e+00   -2.59355e+02   -2.57061e+02   -2.70086e+02
| 5.70900e+00   -2.79251e+02   -2.74051e+02   -2.94808e+02
| 5.80800e+00   -2.99159e+02   -2.91052e+02   -3.19543e+02
| 5.90700e+00   -3.19077e+02   -3.08062e+02   -3.44288e+02
| 6.00600e+00   -3.39003e+02   -3.25080e+02   -3.69042e+02
| 6.10500e+00   -3.58937e+02   -3.42106e+02   -3.93803e+02
| 6.20400e+00   -3.78878e+02   -3.59138e+02   -4.18571e+02
| 6.30300e+00   -3.98826e+02   -3.76177e+02   -4.43346e+02
| 6.40200e+00   -4.18779e+02   -3.93221e+02   -4.68125e+02
| 6.50100e+00   -4.38737e+02   -4.10271e+02   -4.92910e+02
| 6.60000e+00   -4.58699e+02   -4.27325e+02   -5.17700e+02
[Ramp]
|   typ   min   max
dV/dt_r   1.566/0.687n   1.426/0.827n   1.719/0.554n
dV/dt_f   1.396/0.828n   1.212/0.934n   1.595/0.716n
R_load =   50
[Rising Waveform]
R_fixture = 50
V_fixture = 3.3   |Vcc_typ
V_fixture_min = 3.135 |Vcc_min
V_fixture_max = 3.465 |Vcc_max
C_fixture = 0.0p
| Time   typ   min   max
| 0.00000e+00   1.00813e+00   1.14515e+00   8.44568e-01
| 2.69541e-12   1.00813e+00   1.14515e+00   8.44568e-01
| 4.88539e-12   1.00813e+00   1.14515e+00   8.44568e-01
| 5.15560e-12   1.00813e+00   1.14515e+00   8.44568e-01
| 8.43814e-12   1.00813e+00   1.14515e+00   8.44568e-01
| 1.48885e-11   1.00813e+00   1.14515e+00   8.44568e-01
| 1.56443e-11   1.00813e+00   1.14515e+00   8.44568e-01
| 2.89352e-11   1.00813e+00   1.14515e+00   8.44568e-01
| 4.35521e-11   1.00813e+00   1.14515e+00   8.44568e-01
| 4.98146e-11   1.00813e+00   1.14515e+00   8.44568e-01
| 5.87208e-11   1.00813e+00   1.14515e+00   8.44568e-01
| 7.00000e-11   1.00813e+00   1.14515e+00   8.44568e-01
| 7.43355e-11   1.00813e+00   1.14515e+00   8.44568e-01
| 7.98941e-11   1.00813e+00   1.14515e+00   8.44568e-01
| 8.04812e-11   1.00813e+00   1.14515e+00   8.44568e-01
| 8.54765e-11   1.00813e+00   1.14515e+00   8.44568e-01
| 9.54712e-11   1.00813e+00   1.14515e+00   8.44568e-01
| 9.66941e-11   1.00813e+00   1.14515e+00   8.44568e-01
| 1.09694e-10   1.00813e+00   1.14515e+00   8.44568e-01
| 1.16904e-10   1.00813e+00   1.14515e+00   8.44568e-01
| 1.22050e-10   1.00813e+00   1.14515e+00   8.44568e-01
| 1.33756e-10   1.00813e+00   1.14515e+00   8.44568e-01
| 1.42319e-10   1.00813e+00   1.14515e+00   8.44568e-01
| 1.49876e-10   1.00813e+00   1.14515e+00   8.44568e-01
| 1.59675e-10   1.00813e+00   1.14515e+00   8.44568e-01
| 1.71924e-10   1.00813e+00   1.14515e+00   8.44568e-01
| 1.80502e-10   1.00813e+00   1.14515e+00   8.44568e-01
| 1.93342e-10   1.00813e+00   1.14515e+00   8.44568e-01
| 2.03187e-10   1.00813e+00   1.14515e+00   8.44568e-01
| 2.12788e-10   1.00813e+00   1.14515e+00   8.44568e-01
| 2.20117e-10   1.00813e+00   1.14515e+00   8.44568e-01
| 2.25959e-10   1.00813e+00   1.14515e+00   8.44568e-01
| 2.28188e-10   1.00813e+00   1.14515e+00   8.44568e-01
| 2.36412e-10   1.00813e+00   1.14515e+00   8.44568e-01
| 2.43714e-10   1.00813e+00   1.14515e+00   8.44568e-01
| 2.46567e-10   1.00813e+00   1.14515e+00   8.44568e-01
| 2.54564e-10   1.00813e+00   1.14515e+00   8.44568e-01
| 2.64894e-10   1.00813e+00   1.14515e+00   8.44568e-01
| 2.65919e-10   1.00813e+00   1.14515e+00   8.44568e-01
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0s        1.008V     1.145V     844.6mV
41.32ps   1.008V     1.145V     946.4mV
152.4ps   1.065V     1.145V     1.403V
273.9ps   1.466V     1.199V     1.951V
487.3ps   2.198V     1.763V     2.846V
653.1ps   2.706V     2.213V     3.231V
828.8ps   3.044V     2.615V     3.393V
1.094ns   3.242V     2.97V      3.453V
1.505ns   3.294V     3.114V     3.464V
4.666ns   3.3V       3.135V     3.465V
[Falling Waveform]
R_fixture = 50
V_fixture = 3.3   |Vcc_typ
V_fixture_min = 3.135 |Vcc_min
V_fixture_max = 3.465 |Vcc_max
C_fixture = 0.0p
| Time   typ   min   max
| 0.00000e+00   3.30000e+00   3.13500e+00   3.46500e+00
| 2.69541e-12   3.30000e+00   3.13500e+00   3.46500e+00
| 4.88539e-12   3.30000e+00   3.13500e+00   3.46500e+00
| 5.15560e-12   3.30000e+00   3.13500e+00   3.46500e+00
| 8.43814e-12   3.30000e+00   3.13500e+00   3.46500e+00
| 1.48885e-11   3.30000e+00   3.13500e+00   3.46500e+00
| 1.56443e-11   3.30000e+00   3.13500e+00   3.46500e+00
| 2.89352e-11   3.30000e+00   3.13500e+00   3.46500e+00
| 4.35521e-11   3.30000e+00   3.13500e+00   3.46500e+00
| 4.98146e-11   3.30000e+00   3.13500e+00   3.46500e+00
| 5.87207e-11   3.30000e+00   3.13500e+00   3.46500e+00
| 7.00000e-11   3.30000e+00   3.13500e+00   3.46500e+00
| 7.43355e-11   3.30000e+00   3.13500e+00   3.46500e+00
| 7.98941e-11   3.30000e+00   3.13500e+00   3.46500e+00
| 8.04812e-11   3.30000e+00   3.13500e+00   3.46500e+00
| 8.54765e-11   3.30000e+00   3.13500e+00   3.46500e+00
| 9.54712e-11   3.30000e+00   3.13500e+00   3.46500e+00
| 9.66941e-11   3.30000e+00   3.13500e+00   3.46500e+00
| 1.09694e-10   3.30000e+00   3.13500e+00   3.46500e+00
| 1.16904e-10   3.30000e+00   3.13500e+00   3.46500e+00
| 1.22050e-10   3.30000e+00   3.13500e+00   3.46500e+00
| 1.33756e-10   3.30000e+00   3.13500e+00   3.46500e+00
| 1.42318e-10   3.30000e+00   3.13500e+00   3.46500e+00
| 1.49875e-10   3.30000e+00   3.13500e+00   3.46500e+00
| 1.59673e-10   3.30000e+00   3.13500e+00   3.46500e+00
| 1.72937e-10   3.30000e+00   3.13500e+00   3.46500e+00
| 1.80499e-10   3.30000e+00   3.13500e+00   3.46500e+00
| 1.94084e-10   3.30000e+00   3.13500e+00   3.46500e+00
| 2.03953e-10   3.30000e+00   3.13500e+00   3.46500e+00
| 2.17182e-10   3.30000e+00   3.13500e+00   3.46500e+00
| 2.22997e-10   3.30000e+00   3.13500e+00   3.46500e+00
| 2.32435e-10   3.30000e+00   3.13500e+00   3.46500e+00
| 2.41161e-10   3.30000e+00   3.13500e+00   3.46500e+00
| 2.46386e-10   3.30000e+00   3.13500e+00   3.46500e+00
| 2.56120e-10   3.30000e+00   3.13500e+00   3.46500e+00
| 2.57140e-10   3.30000e+00   3.13500e+00   3.46500e+00
| 2.66989e-10   3.30000e+00   3.13500e+00   3.46500e+00
| 2.77410e-10   3.30000e+00   3.13500e+00   3.46500e+00
| 2.83432e-10   3.30000e+00   3.13500e+00   3.46500e+00
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0s        3.3V       3.135V     3.465V
120.1ps   3.304V     3.135V     3.493V
248.1ps   3.333V     3.138V     3.359V
414.7ps   3.222V     3.164V     3.003V
608.4ps   2.915V     3.054V     2.493V
1.058ns   2.032V     2.414V     1.504V
1.49ns    1.442V     1.814V     1.039V
1.93ns    1.159V     1.441V     892.2mV
2.471ns   1.046V     1.24V      853mV
4.662ns   1.008V     1.146V     844.6mV
[Rising Waveform]
R_fixture = 50
V_fixture = 0
C_fixture = 0.0p
| Time   typ   min   max
| 0.00000e+00   2.38922e-08   6.04307e-08   3.04013e-08
| 2.76195e-12   2.38928e-08   6.04313e-08   3.04019e-08
| 5.02196e-12   2.38933e-08   6.04317e-08   3.04024e-08
| 8.43814e-12   2.38939e-08   6.04323e-08   3.04029e-08
| 1.48885e-11   2.38940e-08   6.04329e-08   3.04024e-08
| 2.82261e-11   2.38916e-08   6.04313e-08   3.03997e-08
| 2.96292e-11   2.38914e-08   6.04311e-08   3.03993e-08
| 4.65264e-11   2.38885e-08   6.04278e-08   3.03985e-08
| 5.82632e-11   2.38858e-08   6.04236e-08   3.03966e-08
| 5.99073e-11   2.38849e-08   6.04221e-08   3.03962e-08
| 7.43093e-11   2.38731e-08   6.04054e-08   3.03887e-08
| 7.44096e-11   2.38730e-08   6.04053e-08   3.03887e-08
| 8.01162e-11   2.38724e-08   6.03982e-08   3.03965e-08
| 8.50865e-11   2.38893e-08   6.04041e-08   3.04290e-08
| 8.58855e-11   2.38922e-08   6.04086e-08   3.04412e-08
| 9.61972e-11   2.40299e-08   6.05121e-08   3.05978e-08
| 1.07592e-10   2.42393e-08   6.07310e-08   3.07508e-08
| 1.10532e-10   2.42814e-08   6.07875e-08   3.07286e-08
| 1.20263e-10   2.43167e-08   6.09006e-08   3.05636e-08
| 1.31586e-10   2.39714e-08   6.07198e-08   3.01694e-08
| 1.35499e-10   2.37749e-08   6.06371e-08   2.99415e-08
| 1.46539e-10   2.29494e-08   5.97382e-08   2.91161e-08
| 1.55369e-10   2.17460e-08   5.85776e-08   2.82198e-08
| 1.63542e-10   2.08214e-08   5.72548e-08   2.77165e-08
| 1.77096e-10   1.96382e-08   5.55741e-08   2.77903e-08
| 1.86474e-10   2.06629e-08   5.56641e-08   2.88597e-08
| 1.98457e-10   2.24641e-08   5.66921e-08   3.14336e-08
| 2.09942e-10   2.48232e-08   5.90296e-08   3.38301e-08
| 2.15324e-10   2.58386e-08   6.01251e-08   3.48205e-08
| 2.20167e-10   2.67522e-08   6.09776e-08   3.56009e-08
| 2.27556e-10   2.81662e-08   6.22968e-08   3.65285e-08
| 2.34644e-10   2.94086e-08   6.36264e-08   3.66022e-08
| 2.36605e-10   2.97310e-08   6.40401e-08   3.66226e-08
| 2.44185e-10   3.03322e-08   6.55683e-08   3.54302e-08
| 2.54086e-10   3.02452e-08   6.61629e-08   3.24025e-08
| 2.55652e-10   3.01877e-08   6.60918e-08   3.18819e-08
| 2.65464e-10   2.87003e-08   6.51922e-08   2.86956e-08
| 2.76364e-10   2.59377e-08   6.40738e-08   2.65088e-08
| 2.78193e-10   2.54659e-08   6.38556e-08   2.63593e-08
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0s        23.89nV    60.43nV    30.4nV
197.8ps   -14.21mV   -29.46uV   64.06mV
413.2ps   120.6mV    -13.52mV   649mV
598.4ps   515.1mV    116.9mV    1.273V
889ps     1.248V     622.5mV    2.158V
1.057ns   1.644V     953.2mV    2.489V
1.277ns   2.064V     1.362V     2.703V
1.729ns   2.467V     1.989V     2.821V
2.169ns   2.559V     2.241V     2.839V
4.666ns   2.593V     2.361V     2.845V
[Falling Waveform]
R_fixture = 50
V_fixture = 0
C_fixture = 0.0p
| Time   typ   min   max
| 0.00000e+00   2.59298e+00   2.36182e+00   2.84510e+00
| 7.32301e-10   2.59297e+00   2.36182e+00   2.84511e+00
| 7.45695e-10   2.59297e+00   2.36182e+00   2.84508e+00
| 7.56189e-10   2.59297e+00   2.36182e+00   2.84504e+00
| 7.64187e-10   2.59297e+00   2.36182e+00   2.84501e+00
| 7.77879e-10   2.59298e+00   2.36182e+00   2.84495e+00
| 7.83323e-10   2.59298e+00   2.36182e+00   2.84491e+00
| 7.94399e-10   2.59298e+00   2.36182e+00   2.84473e+00
| 7.99287e-10   2.59298e+00   2.36182e+00   2.84484e+00
| 8.04717e-10   2.59298e+00   2.36182e+00   2.84527e+00
| 8.14850e-10   2.59298e+00   2.36182e+00   2.84672e+00
| 8.19261e-10   2.59298e+00   2.36182e+00   2.84748e+00
| 8.29194e-10   2.59298e+00   2.36182e+00   2.84896e+00
| 8.30494e-10   2.59298e+00   2.36182e+00   2.84911e+00
| 8.41416e-10   2.59297e+00   2.36182e+00   2.84930e+00
| 8.47210e-10   2.59297e+00   2.36182e+00   2.84829e+00
| 8.58620e-10   2.59294e+00   2.36182e+00   2.84243e+00
| 8.62573e-10   2.59293e+00   2.36182e+00   2.83957e+00
| 8.70701e-10   2.59291e+00   2.36182e+00   2.82908e+00
| 8.81144e-10   2.59289e+00   2.36182e+00   2.80718e+00
| 8.90999e-10   2.59287e+00   2.36182e+00   2.77359e+00
| 8.98875e-10   2.59284e+00   2.36182e+00   2.73896e+00
| 9.04944e-10   2.59279e+00   2.36182e+00   2.71078e+00
| 9.10752e-10   2.59276e+00   2.36182e+00   2.68292e+00
| 9.19838e-10   2.59290e+00   2.36182e+00   2.63689e+00
| 9.26265e-10   2.59328e+00   2.36182e+00   2.60403e+00
| 9.31513e-10   2.59376e+00   2.36182e+00   2.57703e+00
| 9.39356e-10   2.59458e+00   2.36181e+00   2.53812e+00
| 9.42788e-10   2.59495e+00   2.36181e+00   2.52109e+00
| 9.52523e-10   2.59582e+00   2.36181e+00   2.47602e+00
| 9.56342e-10   2.59595e+00   2.36180e+00   2.45902e+00
| 9.64820e-10   2.59584e+00   2.36179e+00   2.42164e+00
| 9.70148e-10   2.59508e+00   2.36178e+00   2.39893e+00
| 9.77003e-10   2.59342e+00   2.36177e+00   2.36973e+00
| 9.82632e-10   2.59098e+00   2.36176e+00   2.34587e+00
| 9.88627e-10   2.58750e+00   2.36175e+00   2.32046e+00
| 9.97505e-10   2.57985e+00   2.36174e+00   2.28246e+00
| 1.00365e-09   2.57144e+00   2.36173e+00   2.25617e+00
| 1.01210e-09   2.55514e+00   2.36172e+00   2.21960e+00
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0s        2.593V     2.362V     2.845V
56.92ps   2.593V     2.362V     2.774V
169.6ps   2.571V     2.362V     2.256V
322.8ps   2.013V     2.307V     1.562V
493.7ps   1.382V     1.748V     801.4mV
620.6ps   926.7mV    1.357V     394.7mV
865.1ps   310.3mV    670.1mV    79.39mV
1.091ns   88.07mV    264.7mV    16.51mV
1.468ns   9.955mV    43.91mV    1.142mV
4.662ns   -955.6nV   -1.063uV   -788nV
[Model]   lvcmos_3v3_s10
Model_type   Output
Polarity   Non-Inverting
|   typ   min   max
C_comp   2pF   1.5pF   2.5pF
Vmeas = 1.65V
Rref = 50
Cref = 0
Vref = 1.65V
|   typ   min   max
[Voltage range]   3.3V   3.135V   3.465V
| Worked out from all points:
|   slope of the pulldown table from 0 to 0.495 V, typ, clamps not added: 16.9 ohm
|   slope of the pullup table from 0 to 0.495 V, typ, clamps not added: 12.6 ohm
|   rising waveform, R_fixture 50, V_fixture 3.3: 20-80 % time 424ps typ, 483ps min, 362ps max; typ from 1.01 V to 3.3 V
|   falling waveform, R_fixture 50, V_fixture 3.3: 20-80 % time 794ps typ, 891ps min, 689ps max; typ from 3.3 V to 1.01 V
|   rising waveform, R_fixture 50, V_fixture 0: 20-80 % time 622ps typ, 746ps min, 506ps max; typ from 0 V to 2.59 V
|   falling waveform, R_fixture 50, V_fixture 0: 20-80 % time 438ps typ, 491ps min, 380ps max; typ from 2.59 V to 0 V
[Pulldown]
|Voltage   I (typ)   I (min)   I (max)
|Note, modeling breaks down at 250mA and above.  This is well beyond the functional   |
|operating range of the device.  Should this scenario occur, catastrophic failure and   |
|possible damage to the device and/or board is of higher concern than the I-V curve   |
|behavior.  The IBIS checker will flag currents in excess of 10A with warnings.  Lines   |
|with currents in excess of 0.35 A have been commented out.  The points still remain|
|available to the user if the user desires to use them.   |
|-3.30000e+00   -4.58626e+02   -3.98855e+02   -5.58913e+02
|-3.20100e+00   -4.38670e+02   -3.81813e+02   -5.34126e+02
|-3.10200e+00   -4.18718e+02   -3.64776e+02   -5.09343e+02
|-3.00300e+00   -3.98770e+02   -3.47745e+02   -4.84563e+02
|-2.90400e+00   -3.78827e+02   -3.30720e+02   -4.59787e+02
|-2.80500e+00   -3.58890e+02   -3.13701e+02   -4.35015e+02
|-2.70600e+00   -3.38959e+02   -2.96690e+02   -4.10248e+02
|-2.60700e+00   -3.19035e+02   -2.79688e+02   -3.85486e+02
|-2.50800e+00   -2.99119e+02   -2.62696e+02   -3.60731e+02
|-2.40900e+00   -2.79213e+02   -2.45715e+02   -3.35984e+02
|-2.31000e+00   -2.59319e+02   -2.28747e+02   -3.11245e+02
|-2.21100e+00   -2.39437e+02   -2.11796e+02   -2.86516e+02
|-2.11200e+00   -2.19572e+02   -1.94864e+02   -2.61800e+02
|-2.01300e+00   -1.99726e+02   -1.77955e+02   -2.37100e+02
|-1.91400e+00   -1.79905e+02   -1.61075e+02   -2.12419e+02
|-1.81500e+00   -1.60116e+02   -1.44233e+02   -1.87763e+02
|-1.71600e+00   -1.40369e+02   -1.27441e+02   -1.63140e+02
|-1.61700e+00   -1.20682e+02   -1.10717e+02   -1.38565e+02
|-1.51800e+00   -1.01080e+02   -9.40899e+01   -1.14061e+02
|-1.41900e+00   -8.16135e+01   -7.76121e+01   -8.96701e+01
|-1.32000e+00   -6.23864e+01   -6.13830e+01   -6.54941e+01
|-1.22100e+00   -4.36066e+01   -4.55730e+01   -4.17841e+01
|-1.12200e+00   -2.55446e+01   -3.03740e+01   -1.89497e+01
|-1.02300e+00   -8.13369e+00   -1.57511e+01   -1.01906e+00
|-9.24000e-01   -3.55892e-01   -2.38948e+00   -1.27879e-01
-825mV    -89.74mA   -186.9mA   -97.05mA
-726mV    -64.34mA   -62.46mA   -75.03mA
-627mV    -48.3mA    -42.65mA   -56.86mA
-528mV    -37.22mA   -31.89mA   -45.33mA
363mV     22.88mA    18.45mA    29.33mA
957mV     44.74mA    36.62mA    55.73mA
1.551V    52.05mA    43.3mA     63.04mA
3.531V    55.03mA    47.39mA    66.19mA
3.63V     55.21mA    52.95mA    66.32mA
3.729V    56.59mA    64.36mA    66.46mA
3.828V    63.02mA    84.81mA    66.64mA
3.927V    76.26mA    182.8mA    67.99mA
| 4.02600e+00   9.63336e-02   1.95544e+00   7.56685e-02
| 4.12500e+00   1.29319e-01   1.96109e+01   9.19025e-02
| 4.22400e+00   6.62462e-01   4.21550e+01   1.15435e-01
| 4.32300e+00   1.51637e+01   6.47670e+01   1.37492e-01
| 4.42200e+00   4.22442e+01   8.74545e+01   2.35006e-01
| 4.52100e+00   6.94172e+01   1.10195e+02   8.92943e+00
| 4.62000e+00   9.66780e+01   1.32968e+02   4.35589e+01
| 4.71900e+00   1.23991e+02   1.55761e+02   7.83218e+01
| 4.81800e+00   1.51333e+02   1.78569e+02   1.13180e+02
| 4.91700e+00   1.78693e+02   2.01386e+02   1.48085e+02
| 5.01600e+00   2.06065e+02   2.24210e+02   1.83014e+02
| 5.11500e+00   2.33446e+02   2.47041e+02   2.17958e+02
| 5.21400e+00   2.60834e+02   2.69877e+02   2.52912e+02
| 5.31300e+00   2.88228e+02   2.92717e+02   2.87874e+02
| 5.41200e+00   3.15625e+02   3.15560e+02   3.22841e+02
| 5.51100e+00   3.43027e+02   3.38407e+02   3.57813e+02
| 5.61000e+00   3.70432e+02   3.61256e+02   3.92789e+02
| 5.70900e+00   3.97841e+02   3.84108e+02   4.27769e+02
| 5.80800e+00   4.25252e+02   4.06963e+02   4.62752e+02
| 5.90700e+00   4.52666e+02   4.29821e+02   4.97738e+02
| 6.00600e+00   4.80082e+02   4.52680e+02   5.32727e+02
| 6.10500e+00   5.07501e+02   4.75543e+02   5.67718e+02
| 6.20400e+00   5.34922e+02   4.98407e+02   6.02711e+02
| 6.30300e+00   5.62345e+02   5.21273e+02   6.37705e+02
| 6.40200e+00   5.89770e+02   5.44142e+02   6.72701e+02
| 6.50100e+00   6.17197e+02   5.67013e+02   7.07699e+02
| 6.60000e+00   6.44626e+02   5.89886e+02   7.42698e+02
[Pullup]
|Voltage   I (typ)   I (min)   I (max)
|Note, modeling breaks down at 250mA and above.  This is well beyond the functional   |
|operating range of the device.  Should this scenario occur, catastrophic failure and   |
|possible damage to the device and/or board is of higher concern than the I-V curve   |
|behavior.  The IBIS checker will flag currents in excess of 10A with warnings.  Lines   |
|with currents in excess of 0.35 A have been commented out.  The points still remain|
|available to the user if the user desires to use them.   |
|-3.30000e+00   6.44680e+02   5.51825e+02   8.01095e+02
|-3.20100e+00   6.17254e+02   5.28958e+02   7.66095e+02
|-3.10200e+00   5.89830e+02   5.06093e+02   7.31096e+02
|-3.00300e+00   5.62407e+02   4.83230e+02   6.96098e+02
|-2.90400e+00   5.34987e+02   4.60368e+02   6.61102e+02
|-2.80500e+00   5.07568e+02   4.37509e+02   6.26108e+02
|-2.70600e+00   4.80150e+02   4.14651e+02   5.91115e+02
|-2.60700e+00   4.52735e+02   3.91796e+02   5.56124e+02
|-2.50800e+00   4.25322e+02   3.68942e+02   5.21136e+02
|-2.40900e+00   3.97911e+02   3.46091e+02   4.86149e+02
|-2.31000e+00   3.70503e+02   3.23243e+02   4.51165e+02
|-2.21100e+00   3.43097e+02   3.00397e+02   4.16183e+02
|-2.11200e+00   3.15694e+02   2.77554e+02   3.81204e+02
|-2.01300e+00   2.88295e+02   2.54715e+02   3.46229e+02
|-1.91400e+00   2.60900e+02   2.31881e+02   3.11257e+02
|-1.81500e+00   2.33510e+02   2.09052e+02   2.76290e+02
|-1.71600e+00   2.06127e+02   1.86229e+02   2.41329e+02
|-1.61700e+00   1.78751e+02   1.63415e+02   2.06375e+02
|-1.51800e+00   1.51388e+02   1.40613e+02   1.71432e+02
|-1.41900e+00   1.24042e+02   1.17829e+02   1.36506e+02
|-1.32000e+00   9.67252e+01   9.50724e+01   1.01609e+02
|-1.22100e+00   6.94599e+01   7.23604e+01   6.67700e+01
|-1.12200e+00   4.22820e+01   4.97173e+01   3.20469e+01
|-1.02300e+00   1.51962e+01   2.71494e+01   2.11287e+00
|-9.24000e-01   6.89030e-01   5.34223e+00   1.97623e-01
|-8.25000e-01   1.48916e-01   3.54714e-01   1.54087e-01
-726mV    106.9mA    108.2mA    120.1mA
-627mV    78.63mA    72.64mA    88.74mA
-528mV    57.36mA    52.3mA     65.5mA
-330mV    31.45mA    27.24mA    37.82mA
363mV     -30.02mA   -25.58mA   -36.52mA
957mV     -64.05mA   -54.65mA   -77.43mA
1.353V    -77.99mA   -66.51mA   -94.06mA
1.848V    -87.45mA   -74.38mA   -105.4mA
3.63V     -97.08mA   -83.63mA   -116.9mA
3.729V    -97.47mA   -88.18mA   -117.2mA
3.828V    -98.9mA    -99mA      -117.5mA
3.927V    -104.4mA   -151.4mA   -117.9mA
| 4.02600e+00   -1.15410e-01   -9.65481e-01   -1.19366e-01
| 4.12500e+00   -1.36603e-01   -1.09884e+01   -1.26324e-01
| 4.22400e+00   -3.99361e-01   -2.54841e+01   -1.40663e-01
| 4.32300e+00   -8.17474e+00   -4.04654e+01   -1.58277e-01
| 4.42200e+00   -2.55843e+01   -5.60873e+01   -2.17491e-01
| 4.52100e+00   -4.36450e+01   -7.21990e+01   -4.28595e+00
| 4.62000e+00   -6.24226e+01   -8.86071e+01   -2.64922e+01
| 4.71900e+00   -8.16508e+01   -1.05189e+02   -4.96573e+01
| 4.81800e+00   -1.01115e+02   -1.21884e+02   -7.35635e+01
| 4.91700e+00   -1.20715e+02   -1.38656e+02   -9.78285e+01
| 5.01600e+00   -1.40403e+02   -1.55482e+02   -1.22263e+02
| 5.11500e+00   -1.60149e+02   -1.72350e+02   -1.46794e+02
| 5.21400e+00   -1.79938e+02   -1.89250e+02   -1.71387e+02
| 5.31300e+00   -1.99760e+02   -2.06175e+02   -1.96022e+02
| 5.41200e+00   -2.19606e+02   -2.23121e+02   -2.20688e+02
| 5.51100e+00   -2.39472e+02   -2.40084e+02   -2.45378e+02
| 5.61000e+00   -2.59355e+02   -2.57061e+02   -2.70086e+02
| 5.70900e+00   -2.79251e+02   -2.74051e+02   -2.94808e+02
| 5.80800e+00   -2.99159e+02   -2.91052e+02   -3.19543e+02
| 5.90700e+00   -3.19077e+02   -3.08062e+02   -3.44288e+02
| 6.00600e+00   -3.39003e+02   -3.25080e+02   -3.69042e+02
| 6.10500e+00   -3.58937e+02   -3.42106e+02   -3.93803e+02
| 6.20400e+00   -3.78878e+02   -3.59138e+02   -4.18571e+02
| 6.30300e+00   -3.98826e+02   -3.76177e+02   -4.43346e+02
| 6.40200e+00   -4.18779e+02   -3.93221e+02   -4.68125e+02
| 6.50100e+00   -4.38737e+02   -4.10271e+02   -4.92910e+02
| 6.60000e+00   -4.58699e+02   -4.27325e+02   -5.17700e+02
[Ramp]
|   typ   min   max
dV/dt_r   1.566/0.624n   1.426/0.749n   1.719/0.508n
dV/dt_f   1.396/0.8n   1.212/0.898n   1.595/0.694n
R_load =   50
[Rising Waveform]
R_fixture = 50
V_fixture = 3.3   |Vcc_typ
V_fixture_min = 3.135 |Vcc_min
V_fixture_max = 3.465 |Vcc_max
C_fixture = 0.0p
| Time   typ   min   max
| 0.00000e+00   1.00813e+00   1.14515e+00   8.44568e-01
| 2.69541e-12   1.00813e+00   1.14515e+00   8.44568e-01
| 4.88539e-12   1.00813e+00   1.14515e+00   8.44568e-01
| 5.15560e-12   1.00813e+00   1.14515e+00   8.44568e-01
| 8.43814e-12   1.00813e+00   1.14515e+00   8.44568e-01
| 1.48885e-11   1.00813e+00   1.14515e+00   8.44568e-01
| 1.56443e-11   1.00813e+00   1.14515e+00   8.44568e-01
| 2.89352e-11   1.00813e+00   1.14515e+00   8.44568e-01
| 4.35521e-11   1.00813e+00   1.14515e+00   8.44568e-01
| 4.98146e-11   1.00813e+00   1.14515e+00   8.44568e-01
| 5.87208e-11   1.00813e+00   1.14515e+00   8.44568e-01
| 7.00000e-11   1.00813e+00   1.14515e+00   8.44568e-01
| 7.43355e-11   1.00813e+00   1.14515e+00   8.44568e-01
| 7.98941e-11   1.00813e+00   1.14515e+00   8.44568e-01
| 8.04812e-11   1.00813e+00   1.14515e+00   8.44568e-01
| 8.54765e-11   1.00813e+00   1.14515e+00   8.44568e-01
| 9.54712e-11   1.00813e+00   1.14515e+00   8.44568e-01
| 9.66941e-11   1.00813e+00   1.14515e+00   8.44568e-01
| 1.09694e-10   1.00813e+00   1.14515e+00   8.44568e-01
| 1.16904e-10   1.00813e+00   1.14515e+00   8.44568e-01
| 1.22050e-10   1.00813e+00   1.14515e+00   8.44568e-01
| 1.33756e-10   1.00813e+00   1.14515e+00   8.44568e-01
| 1.42319e-10   1.00813e+00   1.14515e+00   8.44568e-01
| 1.49876e-10   1.00813e+00   1.14515e+00   8.44568e-01
| 1.59675e-10   1.00813e+00   1.14515e+00   8.44568e-01
| 1.71924e-10   1.00813e+00   1.14515e+00   8.44568e-01
| 1.80502e-10   1.00813e+00   1.14515e+00   8.44568e-01
| 1.93342e-10   1.00813e+00   1.14515e+00   8.44568e-01
| 2.03187e-10   1.00813e+00   1.14515e+00   8.44568e-01
| 2.12788e-10   1.00813e+00   1.14515e+00   8.44568e-01
| 2.20117e-10   1.00813e+00   1.14515e+00   8.44568e-01
| 2.25959e-10   1.00813e+00   1.14515e+00   8.44568e-01
| 2.28188e-10   1.00813e+00   1.14515e+00   8.44568e-01
| 2.36412e-10   1.00813e+00   1.14515e+00   8.44568e-01
| 2.43714e-10   1.00813e+00   1.14515e+00   8.44568e-01
| 2.46567e-10   1.00813e+00   1.14515e+00   8.44568e-01
| 2.54564e-10   1.00813e+00   1.14515e+00   8.44568e-01
| 2.64894e-10   1.00813e+00   1.14515e+00   8.44568e-01
| 2.65919e-10   1.00813e+00   1.14515e+00   8.44568e-01
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0s        1.008V     1.145V     844.6mV
41.33ps   1.008V     1.145V     944.7mV
152.4ps   1.064V     1.145V     1.401V
274ps     1.464V     1.198V     1.954V
484.8ps   2.195V     1.755V     2.874V
617.3ps   2.628V     2.117V     3.201V
799ps     3.023V     2.574V     3.388V
1.088ns   3.248V     2.981V     3.455V
1.387ns   3.291V     3.102V     3.463V
4.666ns   3.3V       3.135V     3.465V
[Falling Waveform]
R_fixture = 50
V_fixture = 3.3   |Vcc_typ
V_fixture_min = 3.135 |Vcc_min
V_fixture_max = 3.465 |Vcc_max
C_fixture = 0.0p
| Time   typ   min   max
| 0.00000e+00   3.30000e+00   3.13500e+00   3.46500e+00
| 2.69541e-12   3.30000e+00   3.13500e+00   3.46500e+00
| 4.88539e-12   3.30000e+00   3.13500e+00   3.46500e+00
| 5.15560e-12   3.30000e+00   3.13500e+00   3.46500e+00
| 8.43814e-12   3.30000e+00   3.13500e+00   3.46500e+00
| 1.48885e-11   3.30000e+00   3.13500e+00   3.46500e+00
| 1.56443e-11   3.30000e+00   3.13500e+00   3.46500e+00
| 2.89352e-11   3.30000e+00   3.13500e+00   3.46500e+00
| 4.35521e-11   3.30000e+00   3.13500e+00   3.46500e+00
| 4.98146e-11   3.30000e+00   3.13500e+00   3.46500e+00
| 5.87207e-11   3.30000e+00   3.13500e+00   3.46500e+00
| 7.00000e-11   3.30000e+00   3.13500e+00   3.46500e+00
| 7.43355e-11   3.30000e+00   3.13500e+00   3.46500e+00
| 7.98941e-11   3.30000e+00   3.13500e+00   3.46500e+00
| 8.04812e-11   3.30000e+00   3.13500e+00   3.46500e+00
| 8.54765e-11   3.30000e+00   3.13500e+00   3.46500e+00
| 9.54712e-11   3.30000e+00   3.13500e+00   3.46500e+00
| 9.66941e-11   3.30000e+00   3.13500e+00   3.46500e+00
| 1.09694e-10   3.30000e+00   3.13500e+00   3.46500e+00
| 1.16904e-10   3.30000e+00   3.13500e+00   3.46500e+00
| 1.22050e-10   3.30000e+00   3.13500e+00   3.46500e+00
| 1.33756e-10   3.30000e+00   3.13500e+00   3.46500e+00
| 1.42318e-10   3.30000e+00   3.13500e+00   3.46500e+00
| 1.49875e-10   3.30000e+00   3.13500e+00   3.46500e+00
| 1.59673e-10   3.30000e+00   3.13500e+00   3.46500e+00
| 1.72937e-10   3.30000e+00   3.13500e+00   3.46500e+00
| 1.80499e-10   3.30000e+00   3.13500e+00   3.46500e+00
| 1.94084e-10   3.30000e+00   3.13500e+00   3.46500e+00
| 2.03953e-10   3.30000e+00   3.13500e+00   3.46500e+00
| 2.17182e-10   3.30000e+00   3.13500e+00   3.46500e+00
| 2.22997e-10   3.30000e+00   3.13500e+00   3.46500e+00
| 2.32435e-10   3.30000e+00   3.13500e+00   3.46500e+00
| 2.41161e-10   3.30000e+00   3.13500e+00   3.46500e+00
| 2.46386e-10   3.30000e+00   3.13500e+00   3.46500e+00
| 2.56120e-10   3.30000e+00   3.13500e+00   3.46500e+00
| 2.57140e-10   3.30000e+00   3.13500e+00   3.46500e+00
| 2.66989e-10   3.30000e+00   3.13500e+00   3.46500e+00
| 2.77410e-10   3.30000e+00   3.13500e+00   3.46500e+00
| 2.83432e-10   3.30000e+00   3.13500e+00   3.46500e+00
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0s        3.3V       3.135V     3.465V
119.4ps   3.304V     3.135V     3.493V
222.6ps   3.335V     3.135V     3.382V
385.7ps   3.242V     3.167V     3.024V
575.6ps   2.932V     3.072V     2.5V
986.5ps   2.083V     2.467V     1.552V
1.426ns   1.453V     1.825V     1.047V
1.866ns   1.161V     1.439V     893.2mV
2.346ns   1.052V     1.25V      854.7mV
4.666ns   1.008V     1.146V     844.6mV
[Rising Waveform]
R_fixture = 50
V_fixture = 0
C_fixture = 0.0p
| Time   typ   min   max
| 0.00000e+00   2.38922e-08   6.04307e-08   3.04013e-08
| 2.69541e-12   2.38928e-08   6.04313e-08   3.04019e-08
| 5.02196e-12   2.38933e-08   6.04317e-08   3.04024e-08
| 8.43814e-12   2.38939e-08   6.04323e-08   3.04029e-08
| 1.48885e-11   2.38940e-08   6.04329e-08   3.04024e-08
| 2.82261e-11   2.38916e-08   6.04313e-08   3.03997e-08
| 2.96292e-11   2.38914e-08   6.04311e-08   3.03993e-08
| 4.65264e-11   2.38885e-08   6.04278e-08   3.03985e-08
| 5.82632e-11   2.38858e-08   6.04236e-08   3.03966e-08
| 5.99073e-11   2.38849e-08   6.04221e-08   3.03962e-08
| 7.43093e-11   2.38731e-08   6.04054e-08   3.03887e-08
| 7.44096e-11   2.38730e-08   6.04053e-08   3.03887e-08
| 8.01162e-11   2.38724e-08   6.03982e-08   3.03965e-08
| 8.50865e-11   2.38893e-08   6.04041e-08   3.04290e-08
| 8.58855e-11   2.38922e-08   6.04086e-08   3.04412e-08
| 9.61972e-11   2.40299e-08   6.05121e-08   3.05978e-08
| 1.07592e-10   2.42393e-08   6.07310e-08   3.07508e-08
| 1.10532e-10   2.42814e-08   6.07875e-08   3.07286e-08
| 1.20263e-10   2.43167e-08   6.09006e-08   3.05636e-08
| 1.31586e-10   2.39714e-08   6.07198e-08   3.01694e-08
| 1.35499e-10   2.37749e-08   6.06371e-08   2.99416e-08
| 1.46539e-10   2.29494e-08   5.97382e-08   2.91161e-08
| 1.55369e-10   2.17461e-08   5.85777e-08   2.82199e-08
| 1.63542e-10   2.08216e-08   5.72549e-08   2.77167e-08
| 1.77096e-10   1.96385e-08   5.55744e-08   2.77904e-08
| 1.86474e-10   2.06631e-08   5.56644e-08   2.88598e-08
| 1.98457e-10   2.24642e-08   5.66923e-08   3.14335e-08
| 2.09942e-10   2.48231e-08   5.90296e-08   3.38299e-08
| 2.15324e-10   2.58384e-08   6.01251e-08   3.48203e-08
| 2.20167e-10   2.67520e-08   6.09776e-08   3.56006e-08
| 2.27556e-10   2.81660e-08   6.22967e-08   3.65281e-08
| 2.34644e-10   2.94083e-08   6.36262e-08   3.66019e-08
| 2.36605e-10   2.97306e-08   6.40399e-08   3.66223e-08
| 2.44185e-10   3.03319e-08   6.55680e-08   3.54302e-08
| 2.54086e-10   3.02450e-08   6.61626e-08   3.24026e-08
| 2.55652e-10   3.01875e-08   6.60915e-08   3.18819e-08
| 2.65464e-10   2.87003e-08   6.51920e-08   2.86957e-08
| 2.76364e-10   2.59377e-08   6.40739e-08   2.65089e-08
| 2.78193e-10   2.54660e-08   6.38556e-08   2.63594e-08
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0s        23.89nV    60.43nV    30.4nV
197.9ps   -14.15mV   -25.12uV   64.24mV
412.8ps   122.5mV    -13.73mV   687.4mV
596.4ps   539.2mV    117.2mV    1.366V
834.4ps   1.198V     546.9mV    2.152V
995.7ps   1.623V     892.6mV    2.492V
1.187ns   2.035V     1.295V     2.694V
1.616ns   2.464V     1.976V     2.822V
2.056ns   2.563V     2.251V     2.841V
4.651ns   2.593V     2.361V     2.845V
[Falling Waveform]
R_fixture = 50
V_fixture = 0
C_fixture = 0.0p
| Time   typ   min   max
| 0.00000e+00   2.59298e+00   2.36182e+00   2.84510e+00
| 7.32301e-10   2.59297e+00   2.36182e+00   2.84511e+00
| 7.45695e-10   2.59297e+00   2.36182e+00   2.84508e+00
| 7.56189e-10   2.59297e+00   2.36182e+00   2.84504e+00
| 7.64187e-10   2.59297e+00   2.36182e+00   2.84501e+00
| 7.77879e-10   2.59298e+00   2.36182e+00   2.84495e+00
| 7.83323e-10   2.59298e+00   2.36182e+00   2.84491e+00
| 7.94399e-10   2.59298e+00   2.36182e+00   2.84473e+00
| 7.99287e-10   2.59298e+00   2.36182e+00   2.84484e+00
| 8.04717e-10   2.59298e+00   2.36182e+00   2.84527e+00
| 8.14850e-10   2.59298e+00   2.36182e+00   2.84672e+00
| 8.19260e-10   2.59298e+00   2.36182e+00   2.84748e+00
| 8.29194e-10   2.59298e+00   2.36182e+00   2.84895e+00
| 8.30494e-10   2.59298e+00   2.36182e+00   2.84910e+00
| 8.41399e-10   2.59297e+00   2.36182e+00   2.84929e+00
| 8.47210e-10   2.59297e+00   2.36182e+00   2.84829e+00
| 8.58620e-10   2.59294e+00   2.36182e+00   2.84251e+00
| 8.62522e-10   2.59293e+00   2.36182e+00   2.83974e+00
| 8.70701e-10   2.59291e+00   2.36182e+00   2.82928e+00
| 8.81144e-10   2.59289e+00   2.36182e+00   2.80759e+00
| 8.90957e-10   2.59287e+00   2.36182e+00   2.77444e+00
| 8.98875e-10   2.59284e+00   2.36182e+00   2.73974e+00
| 9.04944e-10   2.59279e+00   2.36182e+00   2.71152e+00
| 9.10693e-10   2.59276e+00   2.36182e+00   2.68391e+00
| 9.19837e-10   2.59290e+00   2.36182e+00   2.63760e+00
| 9.26264e-10   2.59328e+00   2.36182e+00   2.60474e+00
| 9.32010e-10   2.59381e+00   2.36182e+00   2.57518e+00
| 9.39354e-10   2.59458e+00   2.36181e+00   2.53880e+00
| 9.43252e-10   2.59500e+00   2.36181e+00   2.51950e+00
| 9.52521e-10   2.59581e+00   2.36181e+00   2.47657e+00
| 9.56342e-10   2.59594e+00   2.36180e+00   2.45932e+00
| 9.64817e-10   2.59584e+00   2.36179e+00   2.42164e+00
| 9.70148e-10   2.59509e+00   2.36178e+00   2.39842e+00
| 9.77637e-10   2.59326e+00   2.36177e+00   2.36589e+00
| 9.82632e-10   2.59103e+00   2.36176e+00   2.34411e+00
| 9.89303e-10   2.58700e+00   2.36175e+00   2.31503e+00
| 9.97451e-10   2.58007e+00   2.36174e+00   2.27903e+00
| 1.00384e-09   2.57144e+00   2.36173e+00   2.25081e+00
| 1.01210e-09   2.55554e+00   2.36172e+00   2.21383e+00
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0s        2.593V     2.362V     2.845V
56.89ps   2.593V     2.362V     2.774V
169.8ps   2.571V     2.362V     2.251V
322.8ps   2.01V      2.307V     1.528V
553.4ps   1.127V     1.556V     534.1mV
693.5ps   651.3mV    1.113V     222.7mV
827.8ps   337.1mV    724.8mV    89.91mV
1.071ns   87.47mV    264.2mV    16.78mV
1.458ns   9.136mV    41.38mV    1.09mV
4.662ns   -868.1nV   -1.086uV   -705.4nV
